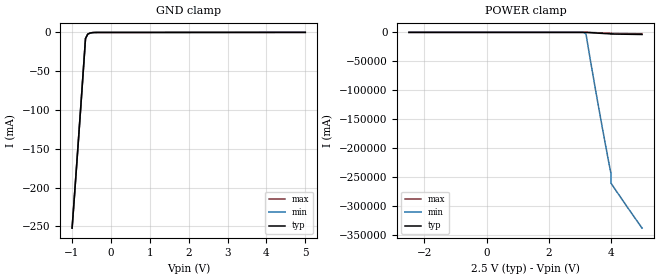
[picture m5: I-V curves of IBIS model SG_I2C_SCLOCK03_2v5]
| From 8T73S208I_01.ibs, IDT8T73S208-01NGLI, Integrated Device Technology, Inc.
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[Model] SG_I2C_SCLOCK03_2v5
Model_type   Input
Polarity   Non-Inverting
Vinl = 0.7V
Vinh = 1.7V
|   typ   min   max
C_comp   2pF   1.5pF   2.5pF
|   typ   min   max
[Voltage range]   2.5V   2.375V   2.625V
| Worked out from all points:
|   GND clamp passes 1 mA (typ) near -0.55 V on its own axis
[GND_clamp]
|Voltage   I (typ)   I (min)   I (max)
-999mV    -252.1mA   -252.1mA   -252.2mA
-826.6mV  -131.9mA   -131.9mA   -131.9mA
-654.2mV  -7.874mA   -7.872mA   -7.877mA
-596.8mV  -2.239mA   -2.236mA   -2.241mA
-481.9mV  -305.7uA   -303.2uA   -308.2uA
-366.9mV  -66.48uA   -64uA      -68.95uA
5V        49.46uA    51.93uA    46.98uA
[Power_clamp]
|Voltage   I (typ)   I (min)   I (max)
-2.5V     49.46uA    49.46uA    49.46uA
3.138V    -5.214mA   -334.8mA   -547.3uA
3.196V    -28.24mA   -3.036A    -1.44mA
3.368V    -622.7mA   -57.79A    -156.3mA
3.598V    -1.388A    -128.3A    -687.1mA
4V        -2.655A    -245A      -1.566A
4.001V    -2.829A    -261A      -1.687A
5V        -3.673A    -338.7A    -2.272A
